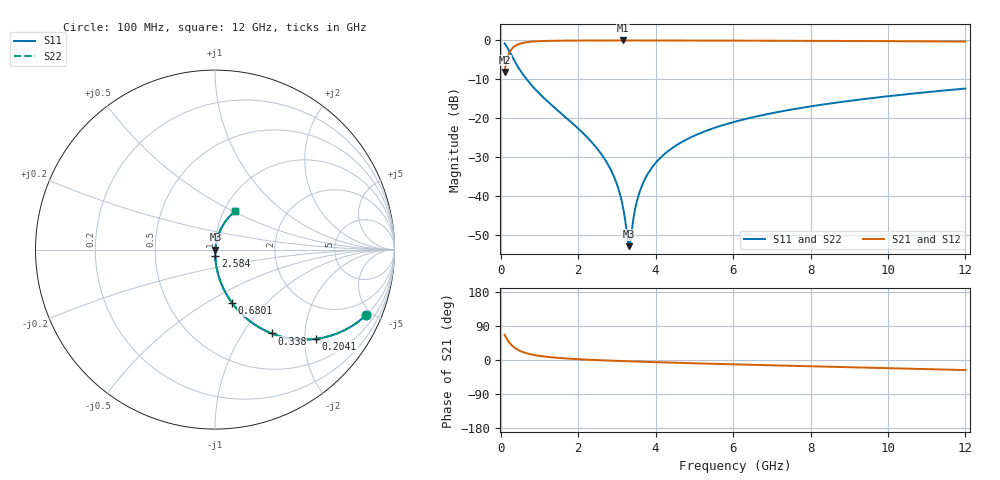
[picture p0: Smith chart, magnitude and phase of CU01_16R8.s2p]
! S-parameter model data by Modelithics Inc. support@modelithics.com 813-866-6335 Tampa FL USA
! S-Parameter data specifications:
! Substrate: 20-mil Rogers, substrate thickness, H=0.508mm, Dielectric constant, Er=3.75
! PCB Mounting Pad Footprint: Pad width, PadW=0.35mm , Pad length, PadL=0.30mm , Pad gap, PadG (edge-to-edge)=0.25mm , Reference planes=0.85mm apart
! Created Tue May  8 14:01:25 2018
# hz S ma R 50
! 2 Port Network Data from SP1.SP block
! freq  magS11  angS11  magS21  angS21  magS12  angS12  magS22  angS22
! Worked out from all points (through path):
!   801 points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, 100 MHz to 12 GHz, reference 50 ohm
!   highest |S21| = -0.02 dB at 3.149 GHz (marker M1); lowest = -8.1 dB at 100 MHz (marker M2)
!   group delay of S21, straight-line fit = 10.3 ps
!   lowest |S11| = -52.8 dB at 3.313 GHz (marker M3), VSWR 1.00, Z = 50.2 - j0.0243 ohm
!   |S11| at or under -10 dB: 670.9 MHz to end of sweep
!   |S22| runs from -52.8 to -0.7 dB; largest |S21 - S12| = 0
!   S11 on the Smith chart (normalised r, x): 100 MHz: 0.99, -4.64; 204.1 MHz: 0.99, -2.27; 338 MHz: 0.99, -1.36; 680.1 MHz: 0.99, -0.65; 2.584 GHz: 1.00, -0.07; 12 GHz: 1.13, +0.51
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1e8  0.9189 -23.3  0.394 66.7  0.394 66.7  0.9189 -23.3
2.04125e8  0.7512 -41.5  0.6594 48.5  0.6594 48.5  0.7512 -41.5
3.38e8  0.5638 -55.9  0.825 34.0  0.825 34.0  0.5638 -55.9
4.8675e8  0.4244 -65.3  0.9044 24.6  0.9044 24.6  0.4244 -65.3
6.80125e8  0.312 -72.3  0.9489 17.5  0.9489 17.5  0.312 -72.3
1.2305e9  0.1613 -81.5  0.9854 8.0  0.9854 8.0  0.1613 -81.5
2.09325e9  0.06693 -86.7  0.9958 1.6  0.9958 1.6  0.06693 -86.7
2.584125e9  0.03551 -87.4  0.9973 -0.7  0.9973 -0.7  0.03551 -87.4
2.92625e9  0.01778 -85.0  0.9976 -2.1  0.9976 -2.1  0.01778 -85.0
3.149375e9  0.007589 -75.7  0.9977 -2.9  0.9977 -2.9  0.007589 -75.7
3.268375e9  0.003041 -44.9  0.9977 -3.3  0.9977 -3.3  0.003041 -44.9
3.313e9  0.002292 -6.1  0.9977 -3.5  0.9977 -3.5  0.002292 -6.1
3.357625e9  0.002913 34.1  0.9976 -3.6  0.9976 -3.6  0.002913 34.1
3.506375e9  0.008248 69.3  0.9976 -4.1  0.9976 -4.1  0.008248 69.3
3.6105e9  0.01228 74.4  0.9975 -4.5  0.9975 -4.5  0.01228 74.4
3.803875e9  0.01962 77.8  0.9973 -5.1  0.9973 -5.1  0.01962 77.8
4.071625e9  0.02934 79.2  0.997 -6.0  0.997 -6.0  0.02934 79.2
4.845125e9  0.05504 79.0  0.9957 -8.2  0.9957 -8.2  0.05504 79.0
6.05e9  0.09056 76.6  0.9928 -11.5  0.9928 -11.5  0.09056 76.6
8.04325e9  0.1433 71.9  0.9861 -16.7  0.9861 -16.7  0.1433 71.9
1.002162e10  0.1926 67.2  0.9772 -21.6  0.9772 -21.6  0.1926 67.2
1.2e10  0.2411 62.4  0.9657 -26.5  0.9657 -26.5  0.2411 62.4
